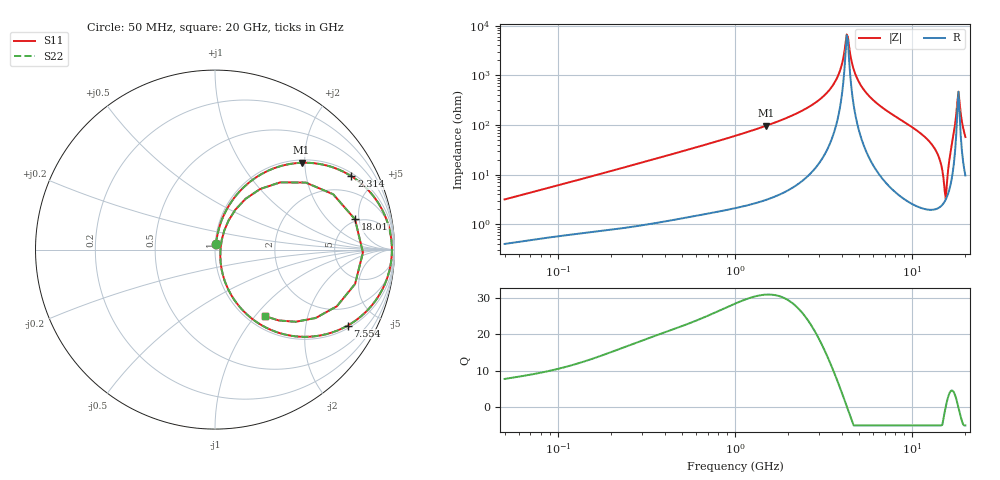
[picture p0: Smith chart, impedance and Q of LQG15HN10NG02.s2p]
!Murata Part Number: LQG15HN10NG02
!These Parameters are Measured in Series Mode Connection
!  o--[Z]--o
!Port1  Port2
!  o-------o
!Freq. Start=50[MHz] Stop=20[GHz], 401[Steps]
# Hz S RI R 50
!Freq.(Hz) S11(Real) S11(Imag) S21(Real) S21(Imag) S12(Real) S12(Imag) S22(Real) S22(Imag)
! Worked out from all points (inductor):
!   401 points, 50 MHz to 20 GHz, reference 50 ohm
!   read as one part in series: L = 9.88 nH near 51.52 MHz
!   highest Q = 31 at 1.498 GHz (marker M1), where L = 10.2 nH
!   self-resonance near 4.276 GHz
!   S11 on the Smith chart (normalised r, x): 50 MHz: 1.01, +0.06; 2.314 GHz: 1.14, +3.64; 7.554 GHz: 1.11, -3.43; 18.01 GHz: 4.72, +4.39; 20 GHz: 1.19, -1.13
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5e7  0.005 0.0312  0.995 -0.0312  0.995 -0.0312  0.005 0.0312
1.364002e8  0.0131 0.0801  0.9869 -0.0801  0.9869 -0.0801  0.0131 0.0801
3.721004e8  0.0548 0.204  0.9452 -0.204  0.9452 -0.204  0.0548 0.204
1e9  0.2731 0.4283  0.7269 -0.4283  0.7269 -0.4283  0.2731 0.4283
1.498439e9  0.4821 0.4838  0.5179 -0.4838  0.5179 -0.4838  0.4821 0.4838
2.313601e9  0.7599 0.4089  0.2401 -0.4089  0.2401 -0.4089  0.7599 0.4089
2.728004e9  0.8545 0.3307  0.1455 -0.3307  0.1455 -0.3307  0.8545 0.3307
3.680849e9  0.9686 0.1264  0.0314 -0.1264  0.0314 -0.1264  0.9686 0.1264
4.275624e9  0.9857 0.00407  0.0143 -0.00407  0.0143 -0.00407  0.9857 0.00407
4.748272e9  0.9784 -0.0846  0.0216 0.0846  0.0216 0.0846  0.9784 -0.0846
5.117541e9  0.963 -0.1477  0.037 0.1477  0.037 0.1477  0.963 -0.1477
7.442007e9  0.7527 -0.4155  0.2473 0.4155  0.2473 0.4155  0.7527 -0.4155
7.554318e9  0.7399 -0.4231  0.2601 0.4231  0.2601 0.4231  0.7399 -0.4231
1.276073e10  0.1669 -0.3508  0.8331 0.3508  0.8331 0.3508  0.1669 -0.3508
1.417136e10  0.0657 -0.204  0.9343 0.204  0.9343 0.204  0.0657 -0.204
1.527346e10  0.0294 -0.0363  0.9706 0.0363  0.9706 0.0363  0.0294 -0.0363
1.573793e10  0.0377 0.0544  0.9623 -0.0544  0.9623 -0.0544  0.0377 0.0544
1.721783e10  0.3641 0.3748  0.6359 -0.3748  0.6359 -0.3748  0.3641 0.3748
1.800918e10  0.7801 0.1689  0.2199 -0.1689  0.2199 -0.1689  0.7801 0.1689
1.855685e10  0.7802 -0.1918  0.2198 0.1918  0.2198 0.1918  0.7802 -0.1918
1.912117e10  0.5606 -0.3812  0.4394 0.3812  0.4394 0.3812  0.5606 -0.3812
2e10  0.2788 -0.371  0.7212 0.371  0.7212 0.371  0.2788 -0.371
